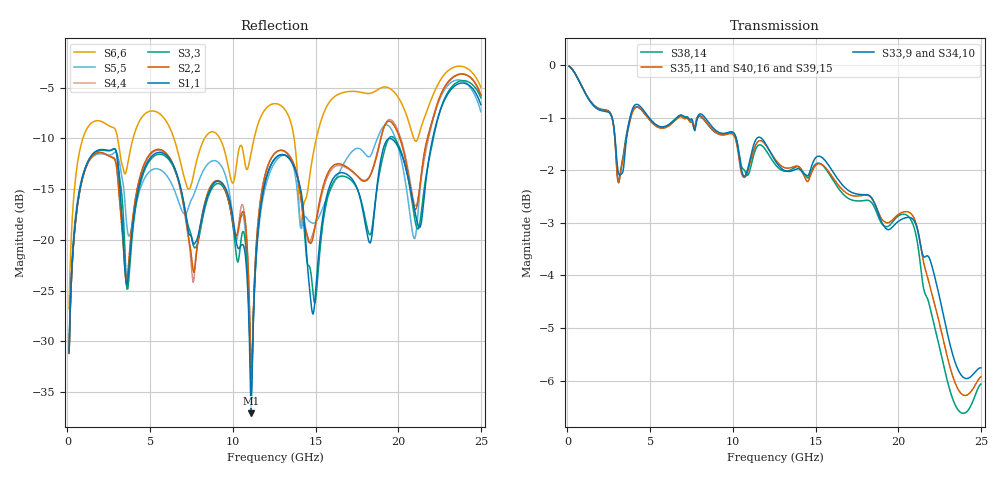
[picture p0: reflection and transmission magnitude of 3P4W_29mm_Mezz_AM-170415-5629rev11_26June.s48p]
! IMPORTANT NOTE: This model should not be used to evaluate
! electrical signals with a greater than 25 GHz. of frequency content.
! Please apply appropriate analysis techniques when reviewing the results of
! your simulations.
!  COPYRIGHT 2008, BY MOLEX INCORPORATED
!  ALL INTERNATIONAL RIGHTS RESERVED
!  THIS FILE CONTAINS MOLEX INCORPORATED CONFIDENTIAL INFORMATION
! >>>>>>>>>>>>>>>>  USER AGREEMENT  <<<<<<<<<<<<<<<<<<<
! The information on this media is the property of MOLEX Incorporated
! and  has been provided to you free of charge. Molex does not
! guarantee that the information is error-free, nor does MOLEX  make
! any representations, warranty or guarantee that the information is
! accurate, correct, reliable or up-to-date. MOLEX expressly
! disclaims all implied warranties regarding this information,
! including but not limited to any implied  warranties of
! merchantability or fitness for a particular purpose. MOLEX does
! not warrant that the media will work correctly in your multi- user
! or network environment.
! MOLEX will in no case be liable for your use, or the results of
! your use, of the software and other information contained on this
! media or  any accompanying written materials.  IT IS YOUR
! RESPONSIBILITY TO VERIFY THE RESULTS OF YOUR USE OF THIS
! INFORMATION IN YOUR OWN PARTICULAR ENGINEERING AND PRODUCT
! ENVIRONMENT, AND YOU ASSUME THE ENTIRE RISK OF DOING SO OR
! FAILING TO DO SO.  In no event will MOLEX be liable for any
! direct, indirect, incidental or consequential damages arising from
! your use of, or your inability to use, software, product simulations
! and other information contained on this media or any accompanying
! written materials.
! This model has not been validated with empirical data.
! This model was solved using HFSS.  TDR results can run 5-8 ohms low
! Touchstone file from project 3P4W_29mm_Mezz_AM-170415-5629rev11_26June
! Exported from HFSS 14.0.0
! Terminal data exported
! Port[1] = B1_T1
! Port[2] = C1_T1
! Port[3] = E1_T1
! Port[4] = F1_T1
! Port[5] = H1_T1
! Port[6] = J1_T1
! Port[7] = A2_T1
! Port[8] = B2_T1
! Port[9] = D2_T1
! Port[10] = E2_T1
! Port[11] = G2_T1
! Port[12] = H2_T1
! Port[13] = B3_T1
! Port[14] = C3_T1
! Port[15] = E3_T1
! Port[16] = F3_T1
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# GHZ S MA R 50.000000
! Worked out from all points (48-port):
!   499 points, 100 MHz to 25 GHz, reference 50 ohm
!   strongest paths, dB at 100 MHz, 6.3 GHz, 12.55 GHz, 18.8 GHz, 25 GHz:
!     S33,9: 0.0, -1.1, -1.8, -2.8, -5.8
!     S34,10: 0.0, -1.1, -1.8, -2.8, -6.0
!     S35,11: 0.0, -1.1, -1.8, -2.8, -5.9
!     S38,14: 0.0, -1.1, -1.9, -2.9, -6.1
!     S40,16: 0.0, -1.1, -1.9, -2.9, -6.1
!     S39,15: 0.0, -1.1, -1.9, -2.8, -6.4
!   lowest |S11| = -37.1 dB at 11.1 GHz (marker M1), VSWR 1.03, Z = 49 - j0.909 ohm
!   |S11| at or under -10 dB: start of sweep to 22.09 GHz
